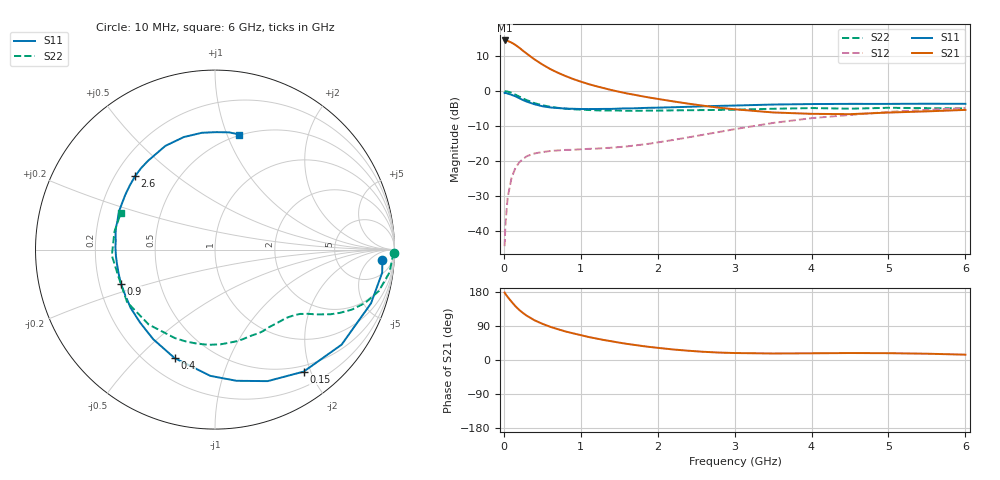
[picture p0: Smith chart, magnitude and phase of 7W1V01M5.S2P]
! Infineon Technologies  Discrete & RF Semiconductors
! BFS17W
! Si NPN RF Bipolar Junction Transistor in SOT323
! VCE = 1 V  IC = 1.5 mA
! Common Emitter S-Parameters:  August  1999
# GHz  S  MA  R  50
!  f  S11  S21  S12  S22
! GHz  MAG  ANG  MAG  ANG  MAG  ANG  MAG  ANG
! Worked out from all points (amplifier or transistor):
!   36 points, 10 MHz to 6 GHz, reference 50 ohm
!   highest |S21| = 14.4 dB at 10 MHz (marker M1)
!   |S21| within 3 dB of that: start of sweep to 252.4 MHz
!   unconditionally stable (mu >= 1): 844.4 MHz to end of sweep
!   at 250 MHz: K = 0.33, MSG = 15.4 dB, |S12| = -19.4 dB
!   at 1.4 GHz: K = 1.39, MAG = 4.5 dB, |S12| = -16.2 dB
!   at 6 GHz: K = 1.13, MAG = -2.5 dB, |S12| = -4.9 dB
!   S11 on the Smith chart (normalised r, x): 10 MHz: 15, -15; 150 MHz: 0.41, -1.89; 400 MHz: 0.31, -0.65; 900 MHz: 0.29, -0.16; 2.6 GHz: 0.28, +0.36; 6 GHz: 0.49, +1.11
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0.01  0.9346 -3.7  5.261 178.0  0.0061 85.8  0.9981 -1.0
0.02  0.9402 -7.9  5.26 174.6  0.0122 85.5  0.989 -2.9
0.05  0.9193 -19.0  5.18 166.3  0.0303 80.0  0.9807 -7.4
0.1  0.8821 -36.9  4.904 153.8  0.0575 69.2  0.9416 -14.2
0.15  0.8402 -54.0  4.543 142.0  0.0795 60.0  0.887 -19.6
0.2  0.7893 -68.2  4.149 132.2  0.0958 53.7  0.8323 -23.7
0.25  0.7407 -80.7  3.742 123.9  0.1073 47.4  0.7795 -26.9
0.3  0.7041 -92.1  3.397 116.6  0.1174 43.2  0.7383 -29.2
0.4  0.6451 -110.4  2.818 104.7  0.1285 37.1  0.6701 -32.6
0.5  0.6064 -124.6  2.392 95.6  0.1343 33.1  0.6266 -34.8
0.6  0.5824 -136.0  2.066 87.8  0.139 31.1  0.5954 -37.0
0.8  0.5607 -153.4  1.637 75.4  0.1442 29.8  0.5598 -41.9
0.9  0.5573 -160.0  1.483 70.4  0.1448 29.7  0.5476 -44.3
1.1  0.552 -171.7  1.256 60.8  0.1494 31.2  0.5351 -49.9
1.6  0.5655 167.0  0.923 42.6  0.1617 38.6  0.5211 -65.9
2.2  0.5858 148.5  0.711 27.8  0.2 47.9  0.5286 -86.6
2.6  0.6047 137.4  0.615 21.6  0.2381 51.2  0.5335 -100.8
3.5  0.6406 115.6  0.494 17.2  0.3499 48.8  0.5574 -131.5
4  0.6507 105.5  0.472 17.7  0.4097 43.6  0.5706 -149.1
4.5  0.655 96.4  0.467 18.4  0.4547 37.9  0.5587 -164.4
5.5  0.6578 83.1  0.512 16.6  0.5369 26.9  0.569 169.9
6  0.6554 78.0  0.537 14.1  0.5694 21.6  0.5634 158.7
